| IBIS file stm32mp157xaa_lfbga448.ibs
[IBIS ver]   4.2
[File name]   stm32mp157xaa_lfbga448.ibs
[File Rev]   2.2
|   rev 2.0: better accuracy
[Date]   07-07-2026
[Source]   Data Created at STMicroelectronics
[Disclaimer]  This information is for modeling purpose only and is
   not guaranted.
   The information is subject to change without notice.
[Copyright]   Copyright 2026 STMicroelectronics Inc.
|   Component stm32mp157xaa_lfbga448
[Component] stm32mp157xaa_lfbga448
[Manufacturer] STMicroelectronics
[Package]
| variable   typ   min   max
R_pkg  6.18E-01  2.42E-01  9.67E-01
L_pkg  3.72E-09  1.45E-09  5.83E-09
C_pkg  1.34E-12  1.04E-12  5.48E-12
[Pin] signal_name model_name
A1 VSS GND
A10 PE3 io8_ft_hslv
A11 PA9 io8_ft_hslv
A12 PB3 io8_ft_hslv
A13 PB14 io8_ft_hslv
A14 VDD POWER
A15 DNU nc
A16 DNU nc
A17 DNU nc
A18 VDD1V2_Unused POWER
A19 VSS GND
A20 DDR_DQ20 PDDRIO_PAD
A21 DDR_DQ23 PDDRIO_PAD
A22 VSS GND
A2 PH5 io8_ft_i2c
A3 PH4 io8_ft_i2c
A4 PE13 io8_ft_hslv
A5 PK6 io8_ft_hslv
A6 PK4 io8_ft
A7 PJ13 io8_ft
A8 PD10 io8_ft_hslv
A9 PD5 io8_ft_hslv
AA1 PG13 io8_ft_hslv_et
AA10 PF7 io8_ft_hslv
AA11 PF6 io8_ft_hslv
AA12 BYPASS_REG1V8 nc
AA13 VSS_USBHS GND
AA14 USB_DM2 nc
AA15 USB_DP1 nc
AA16 VSS_USBHS GND
AA17 USB_RREF POWER
AA18 VSS GND
AA19 DDR_ATO nc
AA20 DDR_DQ29 PDDRIO_PAD
AA21 DDR_DQ28 PDDRIO_PAD
AA22 DDR_DQM3 PDDRIO_PAD
AA2 PG14 io8_ft_hslv_et
AA3 PA0 io8_ft_hslv
AA4 VSS GND
AA5 PB1 io8_ft_hslv
AA6 PC5 io8_ft_hslv
AA7 PB12 io8_ft_hslv_et
AA8 PB5 io8_ft_hslv_et
AA9 PG10 io8_ft_hslv
AB1 VSS GND
AB10 PF8 io8_ft_hslv
AB11 PF9 io8_ft_hslv
AB12 VDDA1V8_REG POWER
AB13 VDD3V3_USBHS POWER
AB14 USB_DP2 nc
AB15 USB_DM1 nc
AB16 VDD3V3_USBFS POWER
AB17 VDDA1V1_REG POWER
AB18 VSS GND
AB19 DDR_VREF POWER
AB20 DDR_DQ27 PDDRIO_PAD
AB21 DDR_DQ26 PDDRIO_PAD
AB22 VSS GND
AB2 PA2 io8_ft_hslv
AB3 PC1 io8_ft_hslv
AB4 PG4 io8_ft_hslv_et
AB5 PB0 io8_ft
AB6 PC4 io8_ft
AB7 PH2 io8_ft_hslv
AB8 PB8 io8_ft_et_i2c_hslv
AB9 PD11 io8_ft_hslv
B1 PH10 io8_ft
B10 PD1 io8_ft_i2c_hslv
B11 PD3 io8_ft_hslv
B12 PB15 io8_ft_hslv
B13 PA8 io8_ft_i2c_hslv
B14 VDDA1V8_Unused POWER
B15 DNU nc
B16 DNU nc
B17 DNU nc
B18 VDD1V2_Unused POWER
B19 VSS GND
B20 DDR_DQ19 PDDRIO_PAD
B21 DDR_DQ16 PDDRIO_PAD
B22 DDR_DQS2N PDIFF_PAD
B2 VSS GND
B3 PH11 io8_ft_i2c
B4 PE14 io8_ft_hslv
B5 PK7 io8_ft
B6 PK3 io8_ft
B7 PJ14 io8_ft
B8 PJ12 io8_ft
B9 PF1 io8_ft_i2c_hslv
C1 PH15 io8_ft
C10 PD0 io8_ft_i2c_hslv
C11 VSS GND
C12 PE5 io8_ft_hslv
C13 PB4 io8_ft_hslv
C14 VSS GND
C15 VSS GND
C16 VSS GND
C17 VSS GND
C18 VSS GND
C19 VSS GND
C20 VSS GND
C21 DDR_DQS2P PDIFF_PAD
C22 DDR_DQM2 PDDRIO_PAD
C2 PH14 io8_ft
C3 VSS GND
C4 PE15 io8_ft
C5 PE0 io8_ft_hslv
C6 PK5 io8_ft_hslv
C7 PJ15 io8_ft
C8 VSS GND
C9 PD4 io8_ft_hslv
D1 PI0 io8_ft
D10 PG15 io8_ft_i2c_hslv
D11 PG6 io8_ft_hslv
D12 PD2 io8_ft_hslv
D13 PC7 io8_ft_hslv
D14 PC9 io8_ft_i2c_hslv
D15 PC11 io8_ft_hslv
D16 JTDI io8_ft
D17 JTCK_SWCLK io8_ft
D18 VDD_PLL2 POWER
D19 VSS_PLL2 GND
D20 DDR_DQ22 PDDRIO_PAD
D21 DDR_DQ17 PDDRIO_PAD
D22 DDR_DQ18 PDDRIO_PAD
D2 PI14 io8_ft_hslv
D3 PH13 io8_ft
D4 VSS GND
D5 PE11 io8_ft
D6 PH8 io8_ft_i2c
D7 PE1 io8_ft
D8 PK0 io8_ft_hslv
D9 PF5 io8_ft_hslv
E1 PI2 io8_ft_hslv
E10 PF0 io8_ft_i2c_hslv
E11 PA15 io8_ft_hslv
E12 PC12 io8_ft_hslv
E13 PC6 io8_ft_hslv
E14 PC8 io8_ft_hslv
E15 NJTRST io8_ft_hslv
E16 JTDO_TRACESWO io8_ft_hslv
E17 JTMS_SWDIO io8_ft_hslv
E18 VDDQ_DDR POWER
E19 VSS GND
E20 DDR_DQ3 PDDRIO_PAD
E21 DDR_DQ0 PDDRIO_PAD
E22 DDR_DQ21 PDDRIO_PAD
E2 PI1 io8_ft_hslv
E3 PI3 io8_ft_hslv
E4 PE12 io8_ft_hslv
E5 VSS GND
E6 PH9 io8_ft
E7 PK1 io8_ft_hslv
E8 PK2 io8_ft_hslv
E9 PE6 io8_ft_hslv
F1 PI7 io8_ft
F10 PD7 io8_ft_i2c_hslv
F11 PB7 io8_ft_i2c_hslv
F12 PB9 io8_ft_i2c_hslv
F13 PF2 io8_ft_hslv
F14 PC10 io8_ft_hslv
F15 PE4 io8_ft_hslv
F16 VSS GND
F17 VDDQ_DDR POWER
F18 DDR_A7 PDDRIO_PAD
F19 DDR_RESETN PDDRIO_PAD
F20 VSS GND
F21 DDR_DQ1 PDDRIO_PAD
F2 PI5 io8_ft
F3 PI15 io8_ft
F4 PZ3 io8_ft_i2c
F5 PH12 io8_ft_i2c
F6 VSS GND
F7 VSS GND
F8 VSS GND
F9 PF4 io8_ft_hslv
G1 PZ4 io8_ft_i2c
G10 VSS GND
G12 VSS GND
G14 VSS GND
G16 VDDQ_DDR POWER
G17 VSS GND
G18 DDR_A13 PDDRIO_PAD
G19 DDR_DQ7 PDDRIO_PAD
G20 DDR_DQM0 PDDRIO_PAD
G21 DDR_DQS0N PDIFF_PAD
G22 DDR_DQS0P PDIFF_PAD
G2 PZ0 io8_ft_i2c_hslv
G3 PZ6 io8_ft_i2c
G4 VSS GND
G5 PI6 io8_ft
G6 VSS GND
G8 VSS GND
H1 PI13 io8_ft_hslv
H11 VDDCORE POWER
H13 VDDCORE POWER
H15 VDDCORE POWER
H17 VDDQ_DDR POWER
H18 DDR_A9 PDDRIO_PAD
H19 DDR_A5 PDDRIO_PAD
H20 DDR_DQ5 PDDRIO_PAD
H21 DDR_DQ2 PDDRIO_PAD
H22 DDR_DQ6 PDDRIO_PAD
H2 PI12 io8_ft_hslv
H3 PZ7 io8_ft_i2c
H4 PZ5 io8_ft_i2c
H5 PZ1 io8_ft_i2c_hslv
H6 PJ8 io8_ft_hslv
H7 VSS GND
H9 VDDCORE POWER
J1 PJ3 io8_ft_hslv
J10 VDDCORE POWER
J11 VSS GND
J12 VDDCORE POWER
J13 VSS GND
J14 VDDCORE POWER
J16 VDDQ_DDR POWER
J17 VSS GND
J18 DDR_A2 PDDRIO_PAD
J19 DDR_A3 PDDRIO_PAD
J20 VSS GND
J21 DDR_DQ4 PDDRIO_PAD
J2 PJ0 io8_ft_hslv
J3 PJ10 io8_ft_hslv
J4 PG12 io8_ft_hslv
J5 PI9 io8_ft
J6 PI4 io8_ft
J8 VDDCORE POWER
J9 VSS GND
K1 PJ5 io8_ft_hslv
K10 VSS GND
K11 VDDCORE POWER
K12 VSS GND
K13 VDDCORE POWER
K14 VSS GND
K15 VDDCORE POWER
K17 VDDQ_DDR POWER
K18 DDR_BA2 PDDRIO_PAD
K19 DDR_A0 PDDRIO_PAD
K20 DDR_BA0 PDDRIO_PAD
K21 DDR_DTO1 PDDRIO_PAD
K22 DDR_ZQ nc
K2 PJ4 io8_ft_hslv
K3 VSS GND
K4 PJ2 io8_ft_hslv
K5 PZ2 io8_ft_i2c_hslv
K6 PJ11 io8_ft_hslv
K7 VSS GND
K9 VDDCORE POWER
L1 PD15 io8_ft
L10 VDDCORE POWER
L11 VSS GND
L12 VDDCORE POWER
L13 VSS GND
L14 VDDCORE POWER
L16 VDDQ_DDR POWER
L17 VSS GND
L18 DDR_CSN PDDRIO_PAD
L19 VSS GND
L20 VSS GND
L21 DDR_ODT PDDRIO_PAD
L22 DDR_DTO0 PDDRIO_PAD
L2 PJ9 io8_ft_hslv
L3 PD6 io8_ft_hslv
L4 PJ7 io8_ft_hslv
L5 PJ6 io8_ft_hslv
L6 PJ1 io8_ft_hslv
L8 VDDCORE POWER
L9 VSS GND
M1 PD8 io8_ft
M10 VSS GND
M11 VDDCORE POWER
M12 VSS GND
M13 VDDCORE POWER
M14 VSS GND
M15 VDDCORE POWER
M17 VDDQ_DDR POWER
M18 DDR_A1 PDDRIO_PAD
M19 DDR_A15 PDDRIO_PAD
M20 DDR_RASN PDDRIO_PAD
M21 DDR_WEN PDDRIO_PAD
M22 DDR_CASN PDDRIO_PAD
M2 PD9 io8_ft
M3 PD14 io8_ft
M4 VBAT POWER
M5 VSS_PLL GND
M6 VDD_PLL POWER
M7 VSS GND
M9 VDD POWER
N1 PI8 io8_ft
N10 VDD POWER
N11 VSS GND
N12 VDDCORE POWER
N13 VSS GND
N14 VDDCORE POWER
N16 VDDQ_DDR POWER
N17 VSS GND
N18 DDR_A10 PDDRIO_PAD
N19 DDR_A12 PDDRIO_PAD
N20 DDR_CLKP PDDRIO_PAD
N21 DDR_CLKN PDDRIO_PAD
N22 DDR_DQ8 PDDRIO_PAD
N2 PC13 io8_ft
N3 BOOT0 io8_ft
N4 BOOT1 io8_ft
N5 VDD_ANA POWER
N6 VREFN GND
N8 VDD POWER
N9 VSS GND
P1 PC14_OSC32_IN io8_ft
P10 VSS GND
P11 VDD POWER
P12 VSS GND
P13 VDDCORE POWER
P14 VSS GND
P15 VDDCORE POWER
P17 VDDQ_DDR POWER
P18 DDR_A14 PDDRIO_PAD
P19 DDR_A11 PDDRIO_PAD
P20 VSS GND
P21 DDR_DQ10 PDDRIO_PAD
P2 PC15_OSC32_OUT io8_ft
P3 VSS GND
P4 BOOT2 io8_ft
P5 VSS_ANA GND
P6 VREF+ POWER
P7 VSS GND
P9 VDD POWER
R1 NRST_CORE isudqf
R10 VDD POWER
R12 VDD POWER
R14 VDDCORE POWER
R16 VDDQ_DDR POWER
R17 VSS GND
R18 DDR_BA1 PDDRIO_PAD
R19 DDR_CKE PDDRIO_PAD
R20 DDR_DQ13 PDDRIO_PAD
R21 DDR_DQ9 PDDRIO_PAD
R22 DDR_DQS1N PDIFF_PAD
|R2 NRST ioreset_ft_v33
R2 NRST nc
R3 PA14 io8_ft
R4 ANA0 nc
R5 VDDA POWER
R6 VSSA GND
R8 VSS GND
T1 PH0_OSC_IN io8_ft
T11 VSS GND
T13 VDD POWER
T15 VDDCORE POWER
T17 VDDQ_DDR POWER
T18 DDR_A4 PDDRIO_PAD
T19 VSS GND
T20 DDR_DQ11 PDDRIO_PAD
T21 DDR_DQM1 PDDRIO_PAD
T22 DDR_DQS1P PDIFF_PAD
T2 PH1_OSC_OUT io8_ft
T3 PI11 io8_ft
T4 PA3 io8_ft
T5 ANA1 nc
T6 VSSA GND
T7 VSS GND
T9 VSS GND
U1 PWR_LP io8_ft
U10 PC0 io8_ft_hslv
U11 PG11 io8_ft_hslv_et
U12 VDD POWER
U13 VSS GND
U14 VDD POWER
U15 VSS GND
U16 VDDQ_DDR POWER
U17 VSS GND
U18 DDR_A8 PDDRIO_PAD
U19 DDR_A6 PDDRIO_PAD
U20 VSS GND
U21 DDR_DQ14 PDDRIO_PAD
U2 PDR_ON_CORE isudqf
U3 PC3 io8_ft_hslv
U4 PG3 io8_ft_hslv_et
U5 PA5 io8_ft_hslv
U6 VSSA GND
U7 VSS GND
U8 PG5 io8_ft
U9 VDD_OTP POWER
V1 PWR_ON io8_ft
V10 PB13 io8_ft_hslv_et
V11 PH6 io8_ft_hslv
V12 PF10 io8_ft_hslv
V13 PB2 io8_ft_hslv
V14 PD13 io8_ft_i2c_hslv
V15 OTG_VBUS io8usb_vbus_otg20_ft
V16 VSS GND
V17 VDDQ_DDR POWER
V18 VSS GND
V19 VSS GND
V20 DDR_DQ12 PDDRIO_PAD
V21 DDR_DQ15 PDDRIO_PAD
V22 DDR_DQ24 PDDRIO_PAD
V2 PDR_ON isudqf
V3 PF3 io8_ft_hslv_et
V4 PA1 io8_ft_hslv
V5 VSS GND
V6 PA4 io8_ft
V7 PF14 io8_ft_i2c_hslv
V8 PF12 io8_ft_hslv
V9 PB10 io8_ft_hslv
W1 PI10 io8_ft
W10 PE7 io8_ft_hslv
W11 PE9 io8_ft_hslv
W12 PD12 io8_ft_i2c_hslv
W13 PB6 io8_ft_i2c_hslv
W14 PE10 io8_ft_hslv
W15 PG9 io8_ft_hslv
W16 PA12 io8_i2c_usb_lsfs_bcd_otg20_ft
W17 VSS GND
W18 VDDQ_DDR POWER
W19 VSS GND
W20 DDR_DQ25 PDDRIO_PAD
W21 DDR_DQ31 PDDRIO_PAD
W22 DDR_DQ30 PDDRIO_PAD
W2 PH7 io8_ft_i2c_hslv
W3 PA13 io8_ft
W4 PG2 io8_ft_hslv_et
W5 PG0 io8_ft_hslv_et
W6 PF15 io8_ft_i2c_hslv
W7 PF13 io8_ft_hslv
W8 PF11 io8_ft_hslv
W9 PA6 io8_ft_hslv
Y1 PC2 io8_ft_hslv_et
Y10 VSS GND
Y11 PG7 io8_ft_hslv
Y12 PE8 io8_ft_hslv
Y13 VSS_USBHS GND
Y14 VSS_USBHS GND
Y15 VSS_USBHS GND
Y16 PA11 io8_i2c_usb_lsfs_bcd_otg20_ft
Y17 PA10 io8usb_id_otg20_ft
Y18 VSS GND
Y19 VDDQ_DDR POWER
Y20 VSS GND
Y21 DDR_DQS3P PDIFF_PAD
Y22 DDR_DQS3N PDIFF_PAD
Y2 PE2 io8_ft_et_i2c_hslv
Y3 VSS GND
Y4 PG1 io8_ft_hslv_et
Y5 PB11 io8_ft_et_i2c_hslv
Y6 PH3 io8_ft_hslv
Y7 VSS GND
Y8 PG8 io8_ft_hslv_et
Y9 PA7 io8_ft_hslv
[Package Model]   500-lfbga-18x18-448-100mhz-181009
[Pin Mapping]   pulldown_ref   pullup_ref   | Comment
A1  VSS  nc
A2  VSS  VDD
A3  VSS  VDD
A4  VSS  VDD
A5  VSS  VDD
A6  VSS  VDD
A7  VSS  VDD
A8  VSS  VDD
A9  VSS  VDD
A10  VSS  VDD
A11  VSS  VDD
A12  VSS  VDD
A13  VSS  VDD
A14  nc  vdd
A15  nc  nc
A16  nc  nc
A17  nc  nc
A18  nc  vdd
A19  VSS  nc
A20  VSS  VDDQ_DDR
A21  VSS  VDDQ_DDR
A22  VSS  nc
AA1  VSS  VDD
AA2  VSS  VDD
AA3  VSS  VDD
AA4  VSS  nc
AA5  VSS  VDD
AA6  VSS  VDD
AA7  VSS  VDD
AA8  VSS  VDD
AA9  VSS  VDD
AA10  VSS  VDD
AA11  VSS  VDD
AA12  nc   nc
AA13  VSS_USBHS  nc
AA14  nc  nc
AA15  nc  nc
AA16  VSS_USBHS  nc
AA17  nc  VDD3V3_USBFS
AA18  VSS  nc
AA19  nc  nc
AA20  VSS  VDDQ_DDR
AA21  VSS  VDDQ_DDR
AA22  VSS  VDDQ_DDR
AB1  VSS  nc
AB2  VSS  VDD
AB3  VSS  VDD
AB4  VSS  VDD
AB5  VSS  VDD
AB6  VSS  VDD
AB7  VSS  VDD
AB8  VSS  VDD
AB9  VSS  VDD
AB10  VSS  VDD
AB11  VSS  VDD
AB12  nc  VDD3V3_USBFS
AB13  nc  vddusbhs
AB14  nc  nc
AB15  nc  nc
AB16  nc  VDD3V3_USBFS
AB17  nc  VDDA1V1_REG
AB18  VSS  nc
AB19  nc   VDDQ_DDR
AB20  VSS  VDDQ_DDR
AB21  VSS  VDDQ_DDR
AB22  VSS  nc
B1  VSS  VDD
B2  VSS  nc
B3  VSS  VDD
B4  VSS  VDD
B5  VSS  VDD
B6  VSS  VDD
B7  VSS  VDD
B8  VSS  VDD
B9  VSS  VDD
B10  VSS  VDD
B11  VSS  VDD
B12  VSS  VDD
B13  VSS  VDD
B14  nc  vdda
B15  nc  nc
B16  nc  nc
B17  nc  nc
B18  nc  VDD1V2_Unused
B19  VSS  nc
B20  VSS  VDDQ_DDR
B21  VSS  VDDQ_DDR
B22  VSS  VDDQ_DDR
C1  VSS  VDD
C2  VSS  VDD
C3  VSS  nc
C4  VSS  VDD
C5  VSS  VDD
C6  VSS  VDD
C7  VSS  VDD
C8  VSS  nc
C9  VSS  VDD
C10  VSS  VDD
C11  VSS  nc
C12  VSS  VDD
C13  VSS  VDD
C14  VSS  nc
C15  VSS  nc
C16  VSS  nc
C17  VSS  nc
C18  VSS  nc
C19  VSS  nc
C20  VSS  nc
C21  VSS  VDDQ_DDR
C22  VSS  VDDQ_DDR
D1  VSS  VDD
D2  VSS  VDD
D3  VSS  VDD
D4  VSS  nc
D5  VSS  VDD
D6  VSS  VDD
D7  VSS  VDD
D8  VSS  VDD
D9  VSS  VDD
D10  VSS  VDD
D11  VSS  VDD
D12  VSS  VDD
D13  VSS  VDD
D14  VSS  VDD
D15  VSS  VDD
D16  VSS  VDD
D17  VSS  VDD
D18  nc  VDD
D19  VSS  nc
D20  VSS  VDDQ_DDR
D21  VSS  VDDQ_DDR
D22  VSS  VDDQ_DDR
E1  VSS  VDD
E2  VSS  VDD
E3  VSS  VDD
E4  VSS  VDD
E5  VSS  nc
E6  VSS  VDD
E7  VSS  VDD
E8  VSS  VDD
E9  VSS  VDD
E10  VSS  VDD
E11  VSS  VDD
E12  VSS  VDD
E13  VSS  VDD
E14  VSS  VDD
E15  VSS  VDD
E16  VSS  VDD
E17  VSS  VDD
E18  nc  VDDQ_DDR
E19  VSS  nc
E20  VSS  VDDQ_DDR
E21  VSS  VDDQ_DDR
E22  VSS  VDDQ_DDR
F1  VSS  VDD
F2  VSS  VDD
F3  VSS  VDD
F4  VSS  VDD
F5  VSS  VDD
F6  VSS  nc
F7  VSS  nc
F8  VSS  nc
F9  VSS  VDD
F10  VSS  VDD
F11  VSS  VDD
F12  VSS  VDD
F13  VSS  VDD
F14  VSS  VDD
F15  VSS  VDD
F16  VSS  nc
F17  nc  VDDQ_DDR
F18  VSS  VDDQ_DDR
F19  VSS  VDDQ_DDR
F20  VSS  nc
F21  VSS  VDDQ_DDR
G1  VSS  VDD
G2  VSS  VDD
G3  VSS  VDD
G4  VSS  nc
G5  VSS  VDD
G6  VSS  nc
G8  VSS  nc
G10  VSS  nc
G12  VSS  nc
G14  VSS  nc
G16  nc  VDDQ_DDR
G17  VSS  nc
G18  VSS  VDDQ_DDR
G19  VSS  VDDQ_DDR
G20  VSS  VDDQ_DDR
G21  VSS  VDDQ_DDR
G22  VSS  VDDQ_DDR
H1  VSS  VDD
H2  VSS  VDD
H3  VSS  VDD
H4  VSS  VDD
H5  VSS  VDD
H6  VSS  VDD
H7  VSS  nc
H9  nc  VDDCORE
H11  nc  VDDCORE
H13  nc  VDDCORE
H15  nc  VDDCORE
H17  nc  VDDQ_DDR
H18  VSS  VDDQ_DDR
H19  VSS  VDDQ_DDR
H20  VSS  VDDQ_DDR
H21  VSS  VDDQ_DDR
H22  VSS  VDDQ_DDR
J1  VSS  VDD
J2  VSS  VDD
J3  VSS  VDD
J4  VSS  VDD
J5  VSS  VDD
J6  VSS  VDD
J8  nc  VDDCORE
J9  VSS  nc
J10  nc  VDDCORE
J11  VSS  nc
J12  nc  VDDCORE
J13  VSS  nc
J14  nc  VDDCORE
J16  nc  VDDQ_DDR
J17  VSS  nc
J18  VSS  VDDQ_DDR
J19  VSS  VDDQ_DDR
J20  VSS  nc
J21  VSS  VDDQ_DDR
K1  VSS  VDD
K2  VSS  VDD
K3  VSS  nc
K4  VSS  VDD
K5  VSS  VDD
K6  VSS  VDD
K7  VSS  nc
K9  nc  VDDCORE
K10  VSS  nc
K11  nc  VDDCORE
K12  VSS  nc
K13  nc  VDDCORE
K14  VSS  nc
K15  nc  VDDCORE
K17  nc  VDDQ_DDR
K18  VSS  VDDQ_DDR
K19  VSS  VDDQ_DDR
K20  VSS  VDDQ_DDR
K21  VSS  VDDQ_DDR
K22  nc  nc
L1  VSS  VDD
L2  VSS  VDD
L3  VSS  VDD
L4  VSS  VDD
L5  VSS  VDD
L6  VSS  VDD
L8  nc  VDDCORE
L9  VSS  nc
L10  nc  VDDCORE
L11  VSS  nc
L12  nc  VDDCORE
L13  VSS  nc
L14  nc  VDDCORE
L16  nc  VDDQ_DDR
L17  VSS  nc
L18  VSS  VDDQ_DDR
L19  VSS  nc
L20  VSS  nc
L21  VSS  VDDQ_DDR
L22  VSS  VDDQ_DDR
M1  VSS  VDD
M2  VSS  VDD
M3  VSS  VDD
M4  nc  VDD_sw
M5  VSS  nc
M6  nc  VDD
M7  VSS  nc
M9  nc  VDD
M10  VSS  nc
M11  nc  VDDCORE
M12  VSS  nc
M13  nc  VDDCORE
M14  VSS  nc
M15  nc  VDDCORE
M17  nc  VDDQ_DDR
M18  VSS  VDDQ_DDR
M19  VSS  VDDQ_DDR
M20  VSS  VDDQ_DDR
M21  VSS  VDDQ_DDR
M22  VSS  VDDQ_DDR
N1  nc  nc
N2  nc  nc
N3  VSS  VDD
N4  VSS  VDD
N5  nc  VDD
N6  VSS  nc
N8  nc  VDD
N9  VSS  nc
N10  nc  VDD
N11  VSS  nc
N12  nc  VDDCORE
N13  VSS  nc
N14  nc  VDDCORE
N16  nc  VDDQ_DDR
N17  VSS  nc
N18  VSS  VDDQ_DDR
N19  VSS  VDDQ_DDR
N20  VSS  VDDQ_DDR
N21  VSS  VDDQ_DDR
N22  VSS  VDDQ_DDR
P1  nc  nc
P2  nc  nc
P3  VSS  nc
P4  VSS  VDD
P5  VSS  nc
P6  nc  VDD
P7  VSS  nc
P9  nc  VDD
P10  VSS  nc
P11  nc  VDD
P12  VSS  nc
P13  nc  VDDCORE
P14  VSS  nc
P15  nc  VDDCORE
P17  nc  VDDQ_DDR
P18  VSS  VDDQ_DDR
P19  VSS  VDDQ_DDR
P20  VSS  nc
P21  VSS  VDDQ_DDR
R1  nc  nc
R2  nc  nc
R3  VSS  VDD
R4  nc  nc
R5  nc  VDD
R6  VSS  nc
R8  VSS  nc
R10  nc  VDD
R12  nc  VDD
R14  nc  VDDCORE
R16  nc  VDDQ_DDR
R17  VSS  nc
R18  VSS  VDDQ_DDR
R19  VSS  VDDQ_DDR
R20  VSS  VDDQ_DDR
R21  VSS  VDDQ_DDR
R22  VSS  VDDQ_DDR
T1  VSS  VDD
T2  VSS  VDD
T3  VSS  VDD
T4  VSS  VDD
T5  nc  nc
T6  VSS  nc
T7  VSS  nc
T9  VSS  nc
T11  VSS  nc
T13  nc  VDD
T15  nc  VDDCORE
T17  nc  VDDQ_DDR
T18  VSS  VDDQ_DDR
T19  VSS  nc
T20  VSS  VDDQ_DDR
T21  VSS  VDDQ_DDR
T22  VSS  VDDQ_DDR
U1  VSS  VDD
U2  nc  nc
U3  VSS  VDD
U4  VSS  VDD
U5  VSS  VDD
U6  VSS  nc
U7  VSS  nc
U8  VSS  VDD
U9  nc  VDD
U10  VSS  VDD
U11  VSS  VDD
U12  nc  VDD
U13  VSS  nc
U14  nc  VDD
U15  VSS  nc
U16  nc  VDDQ_DDR
U17  VSS  nc
U18  VSS  VDDQ_DDR
U19  VSS  VDDQ_DDR
U20  VSS  nc
U21  VSS  VDDQ_DDR
V1  VSS  VDD
V2  nc  nc
V3  VSS  VDD
V4  VSS  VDD
V5  VSS  nc
V6  VSS  VDD
V7  VSS  VDD
V8  VSS  VDD
V9  VSS  VDD
V10  VSS  VDD
V11  VSS  VDD
V12  VSS  VDD
V13  VSS  VDD
V14  VSS  VDD
V15  VSS  VDD3V3_USBFS  | Depending on IO usage
| V15  VSS  VDD  | Depending on IO usage
V16  VSS  nc
V17  nc  VDDQ_DDR
V18  VSS  nc
V19  VSS  nc
V20  VSS  VDDQ_DDR
V21  VSS  VDDQ_DDR
V22  VSS  VDDQ_DDR
W1  VSS  VDD
W2  VSS  VDD
W3  VSS  VDD
W4  VSS  VDD
W5  VSS  VDD
W6  VSS  VDD
W7  VSS  VDD
W8  VSS  VDD
W9  VSS  VDD
W10  VSS  VDD
W11  VSS  VDD
W12  VSS  VDD
W13  VSS  VDD
W14  VSS  VDD
W15  VSS  VDD
W16  VSS  VDD3V3_USBFS  | Depending on IO usage
| W16  VSS  VDD  | Depending on IO usage
W17  VSS  nc
W18  nc  VDDQ_DDR
W19  VSS  nc
W20  VSS  VDDQ_DDR
W21  VSS  VDDQ_DDR
W22  VSS  VDDQ_DDR
Y1  VSS  VDD
Y2  VSS  VDD
Y3  VSS  nc
Y4  VSS  VDD
Y5  VSS  VDD
Y6  VSS  VDD
Y7  VSS  nc
Y8  VSS  VDD
Y9  VSS  VDD
Y10  VSS  nc
Y11  VSS  VDD
Y12  VSS  VDD
Y13  VSS_USBHS  nc
Y14  VSS_USBHS  nc
Y15  VSS_USBHS  nc
Y16  VSS  VDD3V3_USBFS  | Depending on IO usage
| Y16  VSS  VDD  | Depending on IO usage
Y17  VSS  VDD3V3_USBFS  | Depending on IO usage
| Y17  VSS  VDD  | Depending on IO usage
Y18  VSS  nc
Y19  nc  VDDQ_DDR
Y20  VSS  nc
Y21  VSS  VDDQ_DDR
Y22  VSS  VDDQ_DDR
|**********************DIFF PIN*********************************************
[Diff_pin]   inv_pin   vdiff   tdelay_typ   tdelay_min   tdelay_max
   N20   N21   0.320V   0ns   NA   NA   |CK
   G22   G21   0.320V   0ns   NA   NA   |DQS0
   T22   R22   0.320V   0ns   NA   NA   |DQS1
   C21   B22   0.320V   0ns   NA   NA   |DQS2
   Y21   Y22   0.320V   0ns   NA   NA   |DQS3
[Model Selector] io8usb_id_otg20_ft
io8_ft_ls_1v2   "GPIO - 5V tolerant - 1.2V range - Low speed"
io8_ft_ms_1v2   "GPIO - 5V tolerant - 1.2V range - Med speed"
io8_ft_hs_1v2   "GPIO - 5V tolerant - 1.2V range - High speed"
io8_ft_fs_1v2   "GPIO - 5V tolerant - 1.2V range - Fast speed"
io8_ft_hs_1v8   "GPIO - 5V tolerant - 1.8V range - High speed"
io8_ft_fs_1v8   "GPIO - 5V tolerant - 1.8V range - Fast speed"
io8_ft_ms_1v8   "GPIO - 5V tolerant - 1.8V range - Med speed"
io8_ft_ls_1v8   "GPIO - 5V tolerant - 1.8V range - Low speed"
io8_ft_hs_3v3   "GPIO - 5V tolerant - 3.3V range - High speed"
io8_ft_fs_3v3   "GPIO - 5V tolerant - 3.3V range - Fast speed"
io8_ft_ms_3v3   "GPIO - 5V tolerant - 3.3V range - Med speed"
io8_ft_ls_3v3   "GPIO - 5V tolerant - 3.3V range - Low speed"
[Model Selector] io8usb_vbus_otg20_ft
io8_ft_ls_1v2   "GPIO - 5V tolerant - 1.2V range - Low speed"
io8_ft_ms_1v2   "GPIO - 5V tolerant - 1.2V range - Med speed"
io8_ft_hs_1v2   "GPIO - 5V tolerant - 1.2V range - High speed"
io8_ft_fs_1v2   "GPIO - 5V tolerant - 1.2V range - Fast speed"
io8_ft_hs_1v8   "GPIO - 5V tolerant - 1.8V range - High speed"
io8_ft_fs_1v8   "GPIO - 5V tolerant - 1.8V range - Fast speed"
io8_ft_ms_1v8   "GPIO - 5V tolerant - 1.8V range - Med speed"
io8_ft_ls_1v8   "GPIO - 5V tolerant - 1.8V range - Low speed"
io8_ft_hs_3v3   "GPIO - 5V tolerant - 3.3V range - High speed"
io8_ft_fs_3v3   "GPIO - 5V tolerant - 3.3V range - Fast speed"
io8_ft_ms_3v3   "GPIO - 5V tolerant - 3.3V range - Med speed"
io8_ft_ls_3v3   "GPIO - 5V tolerant - 3.3V range - Low speed"
[Model Selector] io8_ft
io8_ft_ls_1v2   "GPIO - 5V tolerant - 1.2V range - Low speed"
io8_ft_ms_1v2   "GPIO - 5V tolerant - 1.2V range - Med speed"
io8_ft_hs_1v2   "GPIO - 5V tolerant - 1.2V range - High speed"
io8_ft_fs_1v2   "GPIO - 5V tolerant - 1.2V range - Fast speed"
io8_ft_hs_1v8   "GPIO - 5V tolerant - 1.8V range - High speed"
io8_ft_fs_1v8   "GPIO - 5V tolerant - 1.8V range - Fast speed"
io8_ft_ms_1v8   "GPIO - 5V tolerant - 1.8V range - Med speed"
io8_ft_ls_1v8   "GPIO - 5V tolerant - 1.8V range - Low speed"
io8_ft_hs_3v3   "GPIO - 5V tolerant - 3.3V range - High speed"
io8_ft_fs_3v3   "GPIO - 5V tolerant - 3.3V range - Fast speed"
io8_ft_ms_3v3   "GPIO - 5V tolerant - 3.3V range - Med speed"
io8_ft_ls_3v3   "GPIO - 5V tolerant - 3.3V range - Low speed"
[Model Selector] io8_ft_hslv
io8_ft_ls_1v2   "GPIO - 5V tolerant - 1.2V range - Low speed"
io8_ft_ms_1v2   "GPIO - 5V tolerant - 1.2V range - Med speed"
io8_ft_hs_1v2   "GPIO - 5V tolerant - 1.2V range - High speed"
io8_ft_fs_1v2   "GPIO - 5V tolerant - 1.2V range - Fast speed"
io8_ft_hs_1v8   "GPIO - 5V tolerant - 1.8V range - High speed"
io8_ft_fs_1v8   "GPIO - 5V tolerant - 1.8V range - Fast speed"
io8_ft_ms_1v8   "GPIO - 5V tolerant - 1.8V range - Med speed"
io8_ft_ls_1v8   "GPIO - 5V tolerant - 1.8V range - Low speed"
io8_ft_hs_3v3   "GPIO - 5V tolerant - 3.3V range - High speed"
io8_ft_fs_3v3   "GPIO - 5V tolerant - 3.3V range - Fast speed"
io8_ft_ms_3v3   "GPIO - 5V tolerant - 3.3V range - Med speed"
io8_ft_ls_3v3   "GPIO - 5V tolerant - 3.3V range - Low speed"
io8_ft_hslv_hs_1v2   "GPIO - hslv opt - 5V tolerant - 1.2V range - High speed"
io8_ft_hslv_fs_1v2   "GPIO - hslv opt - 5V tolerant - 1.2V range - Fast speed"
io8_ft_hslv_ms_1v2   "GPIO - hslv opt - 5V tolerant - 1.2V range - Med speed"
io8_ft_hslv_ls_1v2   "GPIO - hslv opt - 5V tolerant - 1.2V range - Low speed"
io8_ft_hslv_hs_1v8   "GPIO - hslv opt - 5V tolerant - 1.8V range - High speed"
io8_ft_hslv_fs_1v8   "GPIO - hslv opt - 5V tolerant - 1.8V range - Fast speed"
io8_ft_hslv_ms_1v8   "GPIO - hslv opt - 5V tolerant - 1.8V range - Med speed"
io8_ft_hslv_ls_1v8   "GPIO - hslv opt - 5V tolerant - 1.8V range - Low speed"
io8_ft_hslv_hs_2v5   "GPIO - hslv opt - 5V tolerant - 2.5V range - High speed"
io8_ft_hslv_fs_2v5   "GPIO - hslv opt - 5V tolerant - 2.5V range - Fast speed"
io8_ft_hslv_ms_2v5   "GPIO - hslv opt - 5V tolerant - 2.5V range - Med speed"
io8_ft_hslv_ls_2v5   "GPIO - hslv opt - 5V tolerant - 2.5V range - Low speed"
[Model Selector] io8_ft_hslv_et
io8_ft_et_ls_1v2   "GPIO - Ethernet - 5V tol - 1.2V range - Low speed"
io8_ft_et_ms_1v2   "GPIO - Ethernet - 5V tol - 1.2V range - Med speed"
io8_ft_et_hs_1v2   "GPIO - Ethernet - 5V tol - 1.2V range - High speed"
io8_ft_et_fs_1v2   "GPIO - Ethernet - 5V tol - 1.2V range - Fast speed"
io8_ft_et_hs_1v8   "GPIO - Ethernet - 5V tol - 1.8V range - High speed"
io8_ft_et_fs_1v8   "GPIO - Ethernet - 5V tol - 1.8V range - Fast speed"
io8_ft_et_ms_1v8   "GPIO - Ethernet - 5V tol - 1.8V range - Med speed"
io8_ft_et_ls_1v8   "GPIO - Ethernet - 5V tol - 1.8V range - Low speed"
io8_ft_et_hs_3v3   "GPIO - Ethernet - 5V tol - 3.3V range - High speed"
io8_ft_et_fs_3v3   "GPIO - Ethernet - 5V tol - 3.3V range - Fast speed"
io8_ft_et_ms_3v3   "GPIO - Ethernet - 5V tol - 3.3V range - Med speed"
io8_ft_et_ls_3v3   "GPIO - Ethernet - 5V tol - 3.3V range - Low speed"
io8_ft_et_hslv_ls_1v2   "GPIO - hslv opt - Ethernet - 5V tol - 1.2V range - Low speed"
io8_ft_et_hslv_hs_1v2   "GPIO - hslv opt - Ethernet - 5V tol - 1.2V range - High speed"
io8_ft_et_hslv_fs_1v2   "GPIO - hslv opt - Ethernet - 5V tol - 1.2V range - Fast speed"
io8_ft_et_hslv_ms_1v2   "GPIO - hslv opt - Ethernet - 5V tol - 1.2V range - Med speed"
io8_ft_et_hslv_ls_1v8   "GPIO - hslv opt - Ethernet - 5V tol - 1.8V range - Low speed"
io8_ft_et_hslv_hs_1v8   "GPIO - hslv opt - Ethernet - 5V tol - 1.8V range - High speed"
io8_ft_et_hslv_fs_1v8   "GPIO - hslv opt - Ethernet - 5V tol - 1.2V range - Fast speed"
io8_ft_et_hslv_ms_1v8   "GPIO - hslv opt - Ethernet - 5V tol - 1.8V range - Med speed"
io8_ft_et_hslv_hs_2v5   "GPIO - hslv opt - Ethernet - 5V tol - 2.5V range - High speed"
io8_ft_et_hslv_fs_2v5   "GPIO - hslv opt - Ethernet - 5V tol - 2.5V range - Fast speed"
io8_ft_et_hslv_ms_2v5   "GPIO - hslv opt - Ethernet - 5V tol - 2.5V range - Med speed"
io8_ft_et_hslv_ls_2v5   "GPIO - hslv opt - Ethernet - 5V tol - 2.5V range - Low speed"
[Model Selector] io8_ft_et_i2c_hslv
io8_ft_et_ls_1v2   "GPIO - 5V tol - 1.2V range - Low speed"
io8_ft_et_ms_1v2   "GPIO - 5V tol - 1.2V range - Med speed"
io8_ft_et_hs_1v2   "GPIO - 5V tol - 1.2V range - High speed"
io8_ft_et_fs_1v2   "GPIO - 5V tol - 1.2V range - Fast speed"
io8_ft_et_hs_1v8   "GPIO - 5V tol - 1.8V range - High speed"
io8_ft_et_fs_1v8   "GPIO - 5V tol - 1.8V range - Fast speed"
io8_ft_et_ms_1v8   "GPIO - 5V tol - 1.8V range - Med speed"
io8_ft_et_ls_1v8   "GPIO - 5V tol - 1.8V range - Low speed"
io8_ft_et_hs_3v3   "GPIO - 5V tol - 3.3V range - High speed"
io8_ft_et_fs_3v3   "GPIO - 5V tol - 3.3V range - Fast speed"
io8_ft_et_ms_3v3   "GPIO - 5V tol - 3.3V range - Med speed"
io8_ft_et_ls_3v3   "GPIO - 5V tol - 3.3V range - Low speed"
io8_ft_et_hslv_ls_1v2   "GPIO - hslv opt -Ethernet - 5V tol - 1.2V range - Low speed"
io8_ft_et_hslv_hs_1v2   "GPIO - hslv opt -Ethernet - 5V tol - 1.2V range - High speed"
io8_ft_et_hslv_fs_1v2   "GPIO - hslv opt -Ethernet - 5V tol - 1.2V range - Fast speed"
io8_ft_et_hslv_ms_1v2   "GPIO - hslv opt -Ethernet - 5V tol - 1.2V range - Med speed"
io8_ft_et_hslv_ls_1v8   "GPIO - hslv opt -Ethernet - 5V tol - 1.8V range - Low speed"
io8_ft_et_hslv_hs_1v8   "GPIO - hslv opt -Ethernet - 5V tol - 1.8V range - High speed"
io8_ft_et_hslv_fs_1v8   "GPIO - hslv opt -Ethernet - 5V tol - 1.2V range - Fast speed"
io8_ft_et_hslv_ms_1v8   "GPIO - hslv opt -Ethernet - 5V tol - 1.8V range - Med speed"
io8_ft_et_hslv_hs_2v5   "GPIO - hslv opt -Ethernet - 5V tol - 2.5V range - High speed"
io8_ft_et_hslv_fs_2v5   "GPIO - hslv opt  -Ethernet- 5V tol - 2.5V range - Fast speed"
io8_ft_et_hslv_ms_2v5   "GPIO - hslv opt -Ethernet - 5V tol - 2.5V range - Med speed"
io8_ft_et_hslv_ls_2v5   "GPIO - hslv opt -Ethernet - 5V tol - 2.5V range - Low speed"
io8_ft_i2c_1v2   "GPIO - 5V tolerant - 1.2V range - Open drain"
io8_ft_i2c_1v8   "GPIO - 5V tolerant - 1.8V range - Open drain"
io8_ft_i2c_3v3   "GPIO - 5V tolerant - 3.3V range - Open drain"
io8_ft_i2c_hslv_1v2   "GPIO - hslv opt - 5V tolerant - 1.2V range - Open drain"
io8_ft_i2c_hslv_1v8   "GPIO - hslv opt - 5V tolerant - 1.8V range - Open drain"
io8_ft_i2c_hslv_2v5   "GPIO - hslv opt - 5V tolerant - 2.5V range - Open drain"
io8_ft_hslv_hs_1v2   "GPIO - hslv opt - 5V tolerant - 1.2V range - High speed"
io8_ft_hslv_fs_1v2   "GPIO - hslv opt - 5V tolerant - 1.2V range - Fast speed"
io8_ft_hslv_ms_1v2   "GPIO - hslv opt - 5V tolerant - 1.2V range - Med speed"
io8_ft_hslv_ls_1v2   "GPIO - hslv opt - 5V tolerant - 1.2V range - Low speed"
io8_ft_hslv_hs_1v8   "GPIO - hslv opt - 5V tolerant - 1.8V range - High speed"
io8_ft_hslv_fs_1v8   "GPIO - hslv opt - 5V tolerant - 1.8V range - Fast speed"
io8_ft_hslv_ms_1v8   "GPIO - hslv opt - 5V tolerant - 1.8V range - Med speed"
io8_ft_hslv_ls_1v8   "GPIO - hslv opt - 5V tolerant - 1.8V range - Low speed"
io8_ft_hslv_hs_2v5   "GPIO - hslv opt - 5V tolerant - 2.5V range - High speed"
io8_ft_hslv_fs_2v5   "GPIO - hslv opt - 5V tolerant - 2.5V range - Fast speed"
io8_ft_hslv_ms_2v5   "GPIO - hslv opt - 5V tolerant - 2.5V range - Med speed"
io8_ft_hslv_ls_2v5   "GPIO - hslv opt - 5V tolerant - 2.5V range - Low speed"
[Model Selector] io8_ft_i2c
io8_ft_ls_1v2   "GPIO - 5V tolerant - 1.2V range - Low speed"
io8_ft_ms_1v2   "GPIO - 5V tolerant - 1.2V range - Med speed"
io8_ft_hs_1v2   "GPIO - 5V tolerant - 1.2V range - High speed"
io8_ft_fs_1v2   "GPIO - 5V tolerant - 1.2V range - Fast speed"
io8_ft_hs_1v8   "GPIO - 5V tolerant - 1.8V range - High speed"
io8_ft_fs_1v8   "GPIO - 5V tolerant - 1.8V range - Fast speed"
io8_ft_ms_1v8   "GPIO - 5V tolerant - 1.8V range - Med speed"
io8_ft_ls_1v8   "GPIO - 5V tolerant - 1.8V range - Low speed"
io8_ft_hs_3v3   "GPIO - 5V tolerant - 3.3V range - High speed"
io8_ft_fs_3v3   "GPIO - 5V tolerant - 3.3V range - Fast speed"
io8_ft_ms_3v3   "GPIO - 5V tolerant - 3.3V range - Med speed"
io8_ft_ls_3v3   "GPIO - 5V tolerant - 3.3V range - Low speed"
io8_ft_i2c_1v2   "GPIO - 5V tolerant - 1.2V range - Open drain"
io8_ft_i2c_1v8   "GPIO - 5V tolerant - 1.8V range - Open drain"
io8_ft_i2c_3v3   "GPIO - 5V tolerant - 3.3V range - Open drain"
[Model Selector] io8_ft_i2c_hslv
io8_ft_ls_1v2   "GPIO - 5V tolerant - 1.2V range - Low speed"
io8_ft_ms_1v2   "GPIO - 5V tolerant - 1.2V range - Med speed"
io8_ft_hs_1v2   "GPIO - 5V tolerant - 1.2V range - High speed"
io8_ft_fs_1v2   "GPIO - 5V tolerant - 1.2V range - Fast speed"
io8_ft_hs_1v8   "GPIO - 5V tolerant - 1.8V range - High speed"
io8_ft_fs_1v8   "GPIO - 5V tolerant - 1.8V range - Fast speed"
io8_ft_ms_1v8   "GPIO - 5V tolerant - 1.8V range - Med speed"
io8_ft_ls_1v8   "GPIO - 5V tolerant - 1.8V range - Low speed"
io8_ft_hs_3v3   "GPIO - 5V tolerant - 3.3V range - High speed"
io8_ft_fs_3v3   "GPIO - 5V tolerant - 3.3V range - Fast speed"
io8_ft_ms_3v3   "GPIO - 5V tolerant - 3.3V range - Med speed"
io8_ft_ls_3v3   "GPIO - 5V tolerant - 3.3V range - Low speed"
io8_ft_hslv_hs_1v2   "GPIO - hslv opt - 5V tolerant - 1.2V range - High speed"
io8_ft_hslv_fs_1v2   "GPIO - hslv opt - 5V tolerant - 1.2V range - Fast speed"
io8_ft_hslv_ms_1v2   "GPIO - hslv opt - 5V tolerant - 1.2V range - Med speed"
io8_ft_hslv_ls_1v2   "GPIO - hslv opt - 5V tolerant - 1.2V range - Low speed"
io8_ft_hslv_hs_1v8   "GPIO - hslv opt - 5V tolerant - 1.8V range - High speed"
io8_ft_hslv_fs_1v8   "GPIO - hslv opt - 5V tolerant - 1.8V range - Fast speed"
io8_ft_hslv_ms_1v8   "GPIO - hslv opt - 5V tolerant - 1.8V range - Med speed"
io8_ft_hslv_ls_1v8   "GPIO - hslv opt - 5V tolerant - 1.8V range - Low speed"
io8_ft_hslv_hs_2v5   "GPIO - hslv opt - 5V tolerant - 2.5V range - High speed"
io8_ft_hslv_fs_2v5   "GPIO - hslv opt - 5V tolerant - 2.5V range - Fast speed"
io8_ft_hslv_ms_2v5   "GPIO - hslv opt - 5V tolerant - 2.5V range - Med speed"
io8_ft_hslv_ls_2v5   "GPIO - hslv opt - 5V tolerant - 2.5V range - Low speed"
io8_ft_i2c_1v2   "GPIO - 5V tolerant - 1.2V range - Open drain"
io8_ft_i2c_1v8   "GPIO - 5V tolerant - 1.8V range - Open drain"
io8_ft_i2c_3v3   "GPIO - 5V tolerant - 3.3V range - Open drain"
io8_ft_i2c_hslv_1v2   "GPIO - hslv opt - 5V tolerant - 1.2V range - Open drain"
io8_ft_i2c_hslv_1v8   "GPIO - hslv opt - 5V tolerant - 1.8V range - Open drain"
io8_ft_i2c_hslv_2v5   "GPIO - hslv opt - 5V tolerant - 2.5V range - Open drain"
[Model Selector] io8_i2c_usb_lsfs_bcd_otg20_ft
io8_ft_ls_1v2   "GPIO - 5V tolerant - 1.2V range - Low speed"
io8_ft_ms_1v2   "GPIO - 5V tolerant - 1.2V range - Med speed"
io8_ft_hs_1v2   "GPIO - 5V tolerant - 1.2V range - High speed"
io8_ft_fs_1v2   "GPIO - 5V tolerant - 1.2V range - Fast speed"
io8_ft_hs_1v8   "GPIO - 5V tolerant - 1.8V range - High speed"
io8_ft_fs_1v8   "GPIO - 5V tolerant - 1.8V range - Fast speed"
io8_ft_ms_1v8   "GPIO - 5V tolerant - 1.8V range - Med speed"
io8_ft_ls_1v8   "GPIO - 5V tolerant - 1.8V range - Low speed"
io8_ft_hs_3v3   "GPIO - 5V tolerant - 3.3V range - High speed"
io8_ft_fs_3v3   "GPIO - 5V tolerant - 3.3V range - Fast speed"
io8_ft_ms_3v3   "GPIO - 5V tolerant - 3.3V range - Med speed"
io8_ft_ls_3v3   "GPIO - 5V tolerant - 3.3V range - Low speed"
io8_ft_i2c_1v2   "GPIO - 5V tolerant - 1.2V range - Open drain"
io8_ft_i2c_1v8   "GPIO - 5V tolerant - 1.8V range - Open drain"
io8_ft_i2c_3v3   "GPIO - 5V tolerant - 3.3V range - Open drain"
io8usb_ft_hs_3v3   "USB full speed"
io8usb_ft_ls_3v3   "USB low speed"
[Model Selector] isudqf
isudqf_1v2   "Input Buffer - 5V tolerant - 1.2V range"
isudqf_1v8   "Input Buffer - 5V tolerant - 1.8V range"
isudqf_3v3   "Input Buffer - 5V tolerant - 3.3V range"
[Model Selector] PDIFF_PAD
MSD_D3RF2_18   DDR2 MSD_D3R_PDIFF Z0=18-Ohm
MSD_D3RF2_40   DDR2 MSD_D3R_PDIFF Z0=40-Ohm
MSD_D3RF2_48   DDR2 MSD_D3R_PDIFF Z0=48-Ohm
MSD_D3RF2_ODT150   DDR2 MSD_D3R_PDIFF cell 150-Ohm ODT Receiver
MSD_D3RF2_ODT50   DDR2 MSD_D3R_PDIFF cell 50-Ohm ODT Receiver
MSD_D3RF2_ODT75   DDR2 MSD_D3R_PDIFF cell 75-Ohm ODT Receiver
MSD_D3RF2_ODTOFF   DDR2 MSD_D3R_PDIFF cell ODT off Receiver
MSD_D3RF3_34   DDR3 MSD_D3R_PDIFF cell  Z0=34-Ohm
MSD_D3RF3_40   DDR3 MSD_D3R_PDIFF cell  Z0=40-Ohm
MSD_D3RF3_48   DDR3 MSD_D3R_PDIFF cell  Z0=48-Ohm
MSD_D3RF3L_34   DDR3L MSD_D3R_PDIFF cell  Z0=34-Ohm
MSD_D3RF3L_40   DDR3L MSD_D3R_PDIFF cell  Z0=40-Ohm
MSD_D3RF3L_48   DDR3L MSD_D3R_PDIFF cell  Z0=48-Ohm
MSD_D3RF3L_ODT120   DDR3L MSD_D3R_PDIFF cell 120-Ohm ODT Receiver
MSD_D3RF3L_ODT40   DDR3L MSD_D3R_PDIFF cell 40-Ohm ODT Receiver
MSD_D3RF3L_ODT60   DDR3L MSD_D3R_PDIFF cell 60-Ohm ODT Receiver
MSD_D3RF3L_ODTOFF   DDR3L MSD_D3R_PDIFF cell ODT off Receiver
MSD_D3RF3_ODT120   DDR3 MSD_D3R_PDIFF cell 120-Ohm ODT Receiver
MSD_D3RF3_ODT40   DDR3 MSD_D3R_PDIFF cell 40-Ohm ODT Receiver
MSD_D3RF3_ODT60   DDR3 MSD_D3R_PDIFF cell 60-Ohm ODT Receiver
MSD_D3RF3_ODTOFF   DDR3 MSD_D3R_PDIFF cell ODT off Receiver
MSD_D3RFL2_34   LPDDR2 MSD_D3R_PDIFF cell  Z0=34-Ohm
MSD_D3RFL2_40   LPDDR2 MSD_D3R_PDIFF cell  Z0=40-Ohm
MSD_D3RFL2_48   LPDDR2 MSD_D3R_PDIFF cell  Z0=48-Ohm
MSD_D3RFL2_60   LPDDR2 MSD_D3R_PDIFF cell  Z0=60-Ohm
MSD_D3RFL2_80   LPDDR2 MSD_D3R_PDIFF cell  Z0=80-Ohm
MSD_D3RFL2_ODTOFF   LPDDR2 MSD_D3R_PDIFF cell ODT off Receiver
MSD_D3RFL_48   LPDDR MSD_D3R_PDIFF cell  Z0=48-Ohm
MSD_D3RFL_ODTOFF   LPDDR MSD_D3R_PDIFF cell ODT off Receiver
MSD_D3RF2_18_OPEN   DDR2 MSD_D3R_PDIFF_PDQSR Z0=18-Ohm
MSD_D3RF2_40_OPEN   DDR2 MSD_D3R_PDIFF_PDQSR Z0=40-Ohm
MSD_D3RF2_48_OPEN   DDR2 MSD_D3R_PDIFF_PDQSR Z0=48-Ohm
MSD_D3RF2_18_PD344   DDR2 MSD_D3R_PDIFF_PDQSR Z0=18-Ohm
MSD_D3RF2_40_PD344   DDR2 MSD_D3R_PDIFF_PDQSR Z0=40-Ohm
MSD_D3RF2_48_PD344   DDR2 MSD_D3R_PDIFF_PDQSR Z0=48-Ohm
MSD_D3RF2_18_PD393   DDR2 MSD_D3R_PDIFF_PDQSR Z0=18-Ohm
MSD_D3RF2_40_PD393   DDR2 MSD_D3R_PDIFF_PDQSR Z0=40-Ohm
MSD_D3RF2_48_PD393   DDR2 MSD_D3R_PDIFF_PDQSR Z0=48-Ohm
MSD_D3RF2_18_PD458   DDR2 MSD_D3R_PDIFF_PDQSR Z0=18-Ohm
MSD_D3RF2_40_PD458   DDR2 MSD_D3R_PDIFF_PDQSR Z0=40-Ohm
MSD_D3RF2_48_PD458   DDR2 MSD_D3R_PDIFF_PDQSR Z0=48-Ohm
MSD_D3RF2_18_PD500   DDR2 MSD_D3R_PDIFF_PDQSR Z0=18-Ohm
MSD_D3RF2_40_PD500   DDR2 MSD_D3R_PDIFF_PDQSR Z0=40-Ohm
MSD_D3RF2_48_PD500   DDR2 MSD_D3R_PDIFF_PDQSR Z0=48-Ohm
MSD_D3RF2_18_PD550   DDR2 MSD_D3R_PDIFF_PDQSR Z0=18-Ohm
MSD_D3RF2_40_PD550   DDR2 MSD_D3R_PDIFF_PDQSR Z0=40-Ohm
MSD_D3RF2_48_PD550   DDR2 MSD_D3R_PDIFF_PDQSR Z0=48-Ohm
MSD_D3RF2_18_PD611   DDR2 MSD_D3R_PDIFF_PDQSR Z0=18-Ohm
MSD_D3RF2_40_PD611   DDR2 MSD_D3R_PDIFF_PDQSR Z0=40-Ohm
MSD_D3RF2_48_PD611   DDR2 MSD_D3R_PDIFF_PDQSR Z0=48-Ohm
MSD_D3RF2_18_PD688   DDR2 MSD_D3R_PDIFF_PDQSR Z0=18-Ohm
MSD_D3RF2_40_PD688   DDR2 MSD_D3R_PDIFF_PDQSR Z0=40-Ohm
MSD_D3RF2_48_PD688   DDR2 MSD_D3R_PDIFF_PDQSR Z0=48-Ohm
MSD_D3RF2_18_PU344   DDR2 MSD_D3R_PDIFF_PDQSR Z0=18-Ohm
MSD_D3RF2_40_PU344   DDR2 MSD_D3R_PDIFF_PDQSR Z0=40-Ohm
MSD_D3RF2_48_PU344   DDR2 MSD_D3R_PDIFF_PDQSR Z0=48-Ohm
MSD_D3RF2_18_PU393   DDR2 MSD_D3R_PDIFF_PDQSR Z0=18-Ohm
MSD_D3RF2_40_PU393   DDR2 MSD_D3R_PDIFF_PDQSR Z0=40-Ohm
MSD_D3RF2_48_PU393   DDR2 MSD_D3R_PDIFF_PDQSR Z0=48-Ohm
MSD_D3RF2_18_PU458   DDR2 MSD_D3R_PDIFF_PDQSR Z0=18-Ohm
MSD_D3RF2_40_PU458   DDR2 MSD_D3R_PDIFF_PDQSR Z0=40-Ohm
MSD_D3RF2_48_PU458   DDR2 MSD_D3R_PDIFF_PDQSR Z0=48-Ohm
MSD_D3RF2_18_PU500   DDR2 MSD_D3R_PDIFF_PDQSR Z0=18-Ohm
MSD_D3RF2_40_PU500   DDR2 MSD_D3R_PDIFF_PDQSR Z0=40-Ohm
MSD_D3RF2_48_PU500   DDR2 MSD_D3R_PDIFF_PDQSR Z0=48-Ohm
MSD_D3RF2_18_PU550   DDR2 MSD_D3R_PDIFF_PDQSR Z0=18-Ohm
MSD_D3RF2_40_PU550   DDR2 MSD_D3R_PDIFF_PDQSR Z0=40-Ohm
MSD_D3RF2_48_PU550   DDR2 MSD_D3R_PDIFF_PDQSR Z0=48-Ohm
MSD_D3RF2_18_PU611   DDR2 MSD_D3R_PDIFF_PDQSR Z0=18-Ohm
MSD_D3RF2_40_PU611   DDR2 MSD_D3R_PDIFF_PDQSR Z0=40-Ohm
MSD_D3RF2_48_PU611   DDR2 MSD_D3R_PDIFF_PDQSR Z0=48-Ohm
MSD_D3RF2_18_PU688   DDR2 MSD_D3R_PDIFF_PDQSR Z0=18-Ohm
MSD_D3RF2_40_PU688   DDR2 MSD_D3R_PDIFF_PDQSR Z0=40-Ohm
MSD_D3RF2_48_PU688   DDR2 MSD_D3R_PDIFF_PDQSR Z0=48-Ohm
MSD_D3RF2_18_PWRDWN   DDR2 MSD_D3R_PDIFF_PDQSR Z0=18-Ohm
MSD_D3RF2_40_PWRDWN   DDR2 MSD_D3R_PDIFF_PDQSR Z0=40-Ohm
MSD_D3RF2_48_PWRDWN   DDR2 MSD_D3R_PDIFF_PDQSR Z0=48-Ohm
MSD_D3RF3_34_OPEN   DDR3 MSD_D3R_PDIFF_PDQSR cell  Z0=34-Ohm
MSD_D3RF3_40_OPEN   DDR3 MSD_D3R_PDIFF_PDQSR cell  Z0=40-Ohm
MSD_D3RF3_48_OPEN   DDR3 MSD_D3R_PDIFF_PDQSR cell  Z0=48-Ohm
MSD_D3RF3_34_PD344   DDR3 MSD_D3R_PDIFF_PDQSR cell  Z0=34-Ohm
MSD_D3RF3_40_PD344   DDR3 MSD_D3R_PDIFF_PDQSR cell  Z0=40-Ohm
MSD_D3RF3_48_PD344   DDR3 MSD_D3R_PDIFF_PDQSR cell  Z0=48-Ohm
MSD_D3RF3_34_PD393   DDR3 MSD_D3R_PDIFF_PDQSR cell  Z0=34-Ohm
MSD_D3RF3_40_PD393   DDR3 MSD_D3R_PDIFF_PDQSR cell  Z0=40-Ohm
MSD_D3RF3_48_PD393   DDR3 MSD_D3R_PDIFF_PDQSR cell  Z0=48-Ohm
MSD_D3RF3_34_PD458   DDR3 MSD_D3R_PDIFF_PDQSR cell  Z0=34-Ohm
MSD_D3RF3_40_PD458   DDR3 MSD_D3R_PDIFF_PDQSR cell  Z0=40-Ohm
MSD_D3RF3_48_PD458   DDR3 MSD_D3R_PDIFF_PDQSR cell  Z0=48-Ohm
MSD_D3RF3_34_PD500   DDR3 MSD_D3R_PDIFF_PDQSR cell  Z0=34-Ohm
MSD_D3RF3_40_PD500   DDR3 MSD_D3R_PDIFF_PDQSR cell  Z0=40-Ohm
MSD_D3RF3_48_PD500   DDR3 MSD_D3R_PDIFF_PDQSR cell  Z0=48-Ohm
MSD_D3RF3_34_PD550   DDR3 MSD_D3R_PDIFF_PDQSR cell  Z0=34-Ohm
MSD_D3RF3_40_PD550   DDR3 MSD_D3R_PDIFF_PDQSR cell  Z0=40-Ohm
MSD_D3RF3_48_PD550   DDR3 MSD_D3R_PDIFF_PDQSR cell  Z0=48-Ohm
MSD_D3RF3_34_PD611   DDR3 MSD_D3R_PDIFF_PDQSR cell  Z0=34-Ohm
MSD_D3RF3_40_PD611   DDR3 MSD_D3R_PDIFF_PDQSR cell  Z0=40-Ohm
MSD_D3RF3_48_PD611   DDR3 MSD_D3R_PDIFF_PDQSR cell  Z0=48-Ohm
MSD_D3RF3_34_PD688   DDR3 MSD_D3R_PDIFF_PDQSR cell  Z0=34-Ohm
MSD_D3RF3_40_PD688   DDR3 MSD_D3R_PDIFF_PDQSR cell  Z0=40-Ohm
MSD_D3RF3_48_PD688   DDR3 MSD_D3R_PDIFF_PDQSR cell  Z0=48-Ohm
MSD_D3RF3_34_PU344   DDR3 MSD_D3R_PDIFF_PDQSR cell  Z0=34-Ohm
MSD_D3RF3_40_PU344   DDR3 MSD_D3R_PDIFF_PDQSR cell  Z0=40-Ohm
MSD_D3RF3_48_PU344   DDR3 MSD_D3R_PDIFF_PDQSR cell  Z0=48-Ohm
MSD_D3RF3_34_PU393   DDR3 MSD_D3R_PDIFF_PDQSR cell  Z0=34-Ohm
MSD_D3RF3_40_PU393   DDR3 MSD_D3R_PDIFF_PDQSR cell  Z0=40-Ohm
MSD_D3RF3_48_PU393   DDR3 MSD_D3R_PDIFF_PDQSR cell  Z0=48-Ohm
MSD_D3RF3_34_PU458   DDR3 MSD_D3R_PDIFF_PDQSR cell  Z0=34-Ohm
MSD_D3RF3_40_PU458   DDR3 MSD_D3R_PDIFF_PDQSR cell  Z0=40-Ohm
MSD_D3RF3_48_PU458   DDR3 MSD_D3R_PDIFF_PDQSR cell  Z0=48-Ohm
MSD_D3RF3_34_PU500   DDR3 MSD_D3R_PDIFF_PDQSR cell  Z0=34-Ohm
MSD_D3RF3_40_PU500   DDR3 MSD_D3R_PDIFF_PDQSR cell  Z0=40-Ohm
MSD_D3RF3_48_PU500   DDR3 MSD_D3R_PDIFF_PDQSR cell  Z0=48-Ohm
MSD_D3RF3_34_PU550   DDR3 MSD_D3R_PDIFF_PDQSR cell  Z0=34-Ohm
MSD_D3RF3_40_PU550   DDR3 MSD_D3R_PDIFF_PDQSR cell  Z0=40-Ohm
MSD_D3RF3_48_PU550   DDR3 MSD_D3R_PDIFF_PDQSR cell  Z0=48-Ohm
MSD_D3RF3_34_PU611   DDR3 MSD_D3R_PDIFF_PDQSR cell  Z0=34-Ohm
MSD_D3RF3_40_PU611   DDR3 MSD_D3R_PDIFF_PDQSR cell  Z0=40-Ohm
MSD_D3RF3_48_PU611   DDR3 MSD_D3R_PDIFF_PDQSR cell  Z0=48-Ohm
MSD_D3RF3_34_PU688   DDR3 MSD_D3R_PDIFF_PDQSR cell  Z0=34-Ohm
MSD_D3RF3_40_PU688   DDR3 MSD_D3R_PDIFF_PDQSR cell  Z0=40-Ohm
MSD_D3RF3_48_PU688   DDR3 MSD_D3R_PDIFF_PDQSR cell  Z0=48-Ohm
MSD_D3RF3_34_PWRDWN   DDR3 MSD_D3R_PDIFF_PDQSR cell  Z0=34-Ohm
MSD_D3RF3_40_PWRDWN   DDR3 MSD_D3R_PDIFF_PDQSR cell  Z0=40-Ohm
MSD_D3RF3_48_PWRDWN   DDR3 MSD_D3R_PDIFF_PDQSR cell  Z0=48-Ohm
MSD_D3RF3L_34_OPEN   DDR3L MSD_D3R_PDIFF_PDQSR cell  Z0=34-Ohm
MSD_D3RF3L_40_OPEN   DDR3L MSD_D3R_PDIFF_PDQSR cell  Z0=40-Ohm
MSD_D3RF3L_48_OPEN   DDR3L MSD_D3R_PDIFF_PDQSR cell  Z0=48-Ohm
MSD_D3RF3L_34_PD344   DDR3L MSD_D3R_PDIFF_PDQSR cell  Z0=34-Ohm
MSD_D3RF3L_40_PD344   DDR3L MSD_D3R_PDIFF_PDQSR cell  Z0=40-Ohm
MSD_D3RF3L_48_PD344   DDR3L MSD_D3R_PDIFF_PDQSR cell  Z0=48-Ohm
MSD_D3RF3L_34_PD393   DDR3L MSD_D3R_PDIFF_PDQSR cell  Z0=34-Ohm
MSD_D3RF3L_40_PD393   DDR3L MSD_D3R_PDIFF_PDQSR cell  Z0=40-Ohm
MSD_D3RF3L_48_PD393   DDR3L MSD_D3R_PDIFF_PDQSR cell  Z0=48-Ohm
MSD_D3RF3L_34_PD458   DDR3L MSD_D3R_PDIFF_PDQSR cell  Z0=34-Ohm
MSD_D3RF3L_40_PD458   DDR3L MSD_D3R_PDIFF_PDQSR cell  Z0=40-Ohm
MSD_D3RF3L_48_PD458   DDR3L MSD_D3R_PDIFF_PDQSR cell  Z0=48-Ohm
MSD_D3RF3L_34_PD500   DDR3L MSD_D3R_PDIFF_PDQSR cell  Z0=34-Ohm
MSD_D3RF3L_40_PD500   DDR3L MSD_D3R_PDIFF_PDQSR cell  Z0=40-Ohm
MSD_D3RF3L_48_PD500   DDR3L MSD_D3R_PDIFF_PDQSR cell  Z0=48-Ohm
MSD_D3RF3L_34_PD550   DDR3L MSD_D3R_PDIFF_PDQSR cell  Z0=34-Ohm
MSD_D3RF3L_40_PD550   DDR3L MSD_D3R_PDIFF_PDQSR cell  Z0=40-Ohm
MSD_D3RF3L_48_PD550   DDR3L MSD_D3R_PDIFF_PDQSR cell  Z0=48-Ohm
MSD_D3RF3L_34_PD611   DDR3L MSD_D3R_PDIFF_PDQSR cell  Z0=34-Ohm
MSD_D3RF3L_40_PD611   DDR3L MSD_D3R_PDIFF_PDQSR cell  Z0=40-Ohm
MSD_D3RF3L_48_PD611   DDR3L MSD_D3R_PDIFF_PDQSR cell  Z0=48-Ohm
MSD_D3RF3L_34_PD688   DDR3L MSD_D3R_PDIFF_PDQSR cell  Z0=34-Ohm
MSD_D3RF3L_40_PD688   DDR3L MSD_D3R_PDIFF_PDQSR cell  Z0=40-Ohm
MSD_D3RF3L_48_PD688   DDR3L MSD_D3R_PDIFF_PDQSR cell  Z0=48-Ohm
MSD_D3RF3L_34_PU344   DDR3L MSD_D3R_PDIFF_PDQSR cell  Z0=34-Ohm
MSD_D3RF3L_40_PU344   DDR3L MSD_D3R_PDIFF_PDQSR cell  Z0=40-Ohm
MSD_D3RF3L_48_PU344   DDR3L MSD_D3R_PDIFF_PDQSR cell  Z0=48-Ohm
MSD_D3RF3L_34_PU393   DDR3L MSD_D3R_PDIFF_PDQSR cell  Z0=34-Ohm
MSD_D3RF3L_40_PU393   DDR3L MSD_D3R_PDIFF_PDQSR cell  Z0=40-Ohm
MSD_D3RF3L_48_PU393   DDR3L MSD_D3R_PDIFF_PDQSR cell  Z0=48-Ohm
MSD_D3RF3L_34_PU458   DDR3L MSD_D3R_PDIFF_PDQSR cell  Z0=34-Ohm
MSD_D3RF3L_40_PU458   DDR3L MSD_D3R_PDIFF_PDQSR cell  Z0=40-Ohm
MSD_D3RF3L_48_PU458   DDR3L MSD_D3R_PDIFF_PDQSR cell  Z0=48-Ohm
MSD_D3RF3L_34_PU500   DDR3L MSD_D3R_PDIFF_PDQSR cell  Z0=34-Ohm
MSD_D3RF3L_40_PU500   DDR3L MSD_D3R_PDIFF_PDQSR cell  Z0=40-Ohm
MSD_D3RF3L_48_PU500   DDR3L MSD_D3R_PDIFF_PDQSR cell  Z0=48-Ohm
MSD_D3RF3L_34_PU550   DDR3L MSD_D3R_PDIFF_PDQSR cell  Z0=34-Ohm
MSD_D3RF3L_40_PU550   DDR3L MSD_D3R_PDIFF_PDQSR cell  Z0=40-Ohm
MSD_D3RF3L_48_PU550   DDR3L MSD_D3R_PDIFF_PDQSR cell  Z0=48-Ohm
MSD_D3RF3L_34_PU611   DDR3L MSD_D3R_PDIFF_PDQSR cell  Z0=34-Ohm
MSD_D3RF3L_40_PU611   DDR3L MSD_D3R_PDIFF_PDQSR cell  Z0=40-Ohm
MSD_D3RF3L_48_PU611   DDR3L MSD_D3R_PDIFF_PDQSR cell  Z0=48-Ohm
MSD_D3RF3L_34_PU688   DDR3L MSD_D3R_PDIFF_PDQSR cell  Z0=34-Ohm
MSD_D3RF3L_40_PU688   DDR3L MSD_D3R_PDIFF_PDQSR cell  Z0=40-Ohm
MSD_D3RF3L_48_PU688   DDR3L MSD_D3R_PDIFF_PDQSR cell  Z0=48-Ohm
MSD_D3RF3L_34_PWRDWN   DDR3L MSD_D3R_PDIFF_PDQSR cell  Z0=34-Ohm
MSD_D3RF3L_40_PWRDWN   DDR3L MSD_D3R_PDIFF_PDQSR cell  Z0=40-Ohm
MSD_D3RF3L_48_PWRDWN   DDR3L MSD_D3R_PDIFF_PDQSR cell  Z0=48-Ohm
MSD_D3RFL2_34_OPEN   LPDDR2 MSD_D3R_PDIFF_PDQSR cell  Z0=34-Ohm
MSD_D3RFL2_40_OPEN   LPDDR2 MSD_D3R_PDIFF_PDQSR cell  Z0=40-Ohm
MSD_D3RFL2_48_OPEN   LPDDR2 MSD_D3R_PDIFF_PDQSR cell  Z0=48-Ohm
MSD_D3RFL2_60_OPEN   LPDDR2 MSD_D3R_PDIFF_PDQSR cell  Z0=60-Ohm
MSD_D3RFL2_80_OPEN   LPDDR2 MSD_D3R_PDIFF_PDQSR cell  Z0=80-Ohm
MSD_D3RFL_48_OPEN   LPDDR MSD_D3R_PDIFF_PDQSR cell  Z0=48-Ohm
MSD_D3RFL2_34_PD344   LPDDR2 MSD_D3R_PDIFF_PDQSR cell  Z0=34-Ohm
MSD_D3RFL2_40_PD344   LPDDR2 MSD_D3R_PDIFF_PDQSR cell  Z0=40-Ohm
MSD_D3RFL2_48_PD344   LPDDR2 MSD_D3R_PDIFF_PDQSR cell  Z0=48-Ohm
MSD_D3RFL2_60_PD344   LPDDR2 MSD_D3R_PDIFF_PDQSR cell  Z0=60-Ohm
MSD_D3RFL2_80_PD344   LPDDR2 MSD_D3R_PDIFF_PDQSR cell  Z0=80-Ohm
MSD_D3RFL_48_PD344   LPDDR MSD_D3R_PDIFF_PDQSR cell  Z0=48-Ohm
MSD_D3RFL2_34_PD393   LPDDR2 MSD_D3R_PDIFF_PDQSR cell  Z0=34-Ohm
MSD_D3RFL2_40_PD393   LPDDR2 MSD_D3R_PDIFF_PDQSR cell  Z0=40-Ohm
MSD_D3RFL2_48_PD393   LPDDR2 MSD_D3R_PDIFF_PDQSR cell  Z0=48-Ohm
MSD_D3RFL2_60_PD393   LPDDR2 MSD_D3R_PDIFF_PDQSR cell  Z0=60-Ohm
MSD_D3RFL2_80_PD393   LPDDR2 MSD_D3R_PDIFF_PDQSR cell  Z0=80-Ohm
MSD_D3RFL_48_PD393   LPDDR MSD_D3R_PDIFF_PDQSR cell  Z0=48-Ohm
MSD_D3RFL2_34_PD458   LPDDR2 MSD_D3R_PDIFF_PDQSR cell  Z0=34-Ohm
MSD_D3RFL2_40_PD458   LPDDR2 MSD_D3R_PDIFF_PDQSR cell  Z0=40-Ohm
MSD_D3RFL2_48_PD458   LPDDR2 MSD_D3R_PDIFF_PDQSR cell  Z0=48-Ohm
MSD_D3RFL2_60_PD458   LPDDR2 MSD_D3R_PDIFF_PDQSR cell  Z0=60-Ohm
MSD_D3RFL2_80_PD458   LPDDR2 MSD_D3R_PDIFF_PDQSR cell  Z0=80-Ohm
MSD_D3RFL_48_PD458   LPDDR MSD_D3R_PDIFF_PDQSR cell  Z0=48-Ohm
MSD_D3RFL2_34_PD500   LPDDR2 MSD_D3R_PDIFF_PDQSR cell  Z0=34-Ohm
MSD_D3RFL2_40_PD500   LPDDR2 MSD_D3R_PDIFF_PDQSR cell  Z0=40-Ohm
MSD_D3RFL2_48_PD500   LPDDR2 MSD_D3R_PDIFF_PDQSR cell  Z0=48-Ohm
MSD_D3RFL2_60_PD500   LPDDR2 MSD_D3R_PDIFF_PDQSR cell  Z0=60-Ohm
MSD_D3RFL2_80_PD500   LPDDR2 MSD_D3R_PDIFF_PDQSR cell  Z0=80-Ohm
MSD_D3RFL_48_PD500   LPDDR MSD_D3R_PDIFF_PDQSR cell  Z0=48-Ohm
MSD_D3RFL2_34_PD550   LPDDR2 MSD_D3R_PDIFF_PDQSR cell  Z0=34-Ohm
MSD_D3RFL2_40_PD550   LPDDR2 MSD_D3R_PDIFF_PDQSR cell  Z0=40-Ohm
MSD_D3RFL2_48_PD550   LPDDR2 MSD_D3R_PDIFF_PDQSR cell  Z0=48-Ohm
MSD_D3RFL2_60_PD550   LPDDR2 MSD_D3R_PDIFF_PDQSR cell  Z0=60-Ohm
MSD_D3RFL2_80_PD550   LPDDR2 MSD_D3R_PDIFF_PDQSR cell  Z0=80-Ohm
MSD_D3RFL_48_PD550   LPDDR MSD_D3R_PDIFF_PDQSR cell  Z0=48-Ohm
MSD_D3RFL2_34_PD611   LPDDR2 MSD_D3R_PDIFF_PDQSR cell  Z0=34-Ohm
MSD_D3RFL2_40_PD611   LPDDR2 MSD_D3R_PDIFF_PDQSR cell  Z0=40-Ohm
MSD_D3RFL2_48_PD611   LPDDR2 MSD_D3R_PDIFF_PDQSR cell  Z0=48-Ohm
MSD_D3RFL2_60_PD611   LPDDR2 MSD_D3R_PDIFF_PDQSR cell  Z0=60-Ohm
MSD_D3RFL2_80_PD611   LPDDR2 MSD_D3R_PDIFF_PDQSR cell  Z0=80-Ohm
MSD_D3RFL_48_PD611   LPDDR MSD_D3R_PDIFF_PDQSR cell  Z0=48-Ohm
MSD_D3RFL2_34_PD688   LPDDR2 MSD_D3R_PDIFF_PDQSR cell  Z0=34-Ohm
MSD_D3RFL2_40_PD688   LPDDR2 MSD_D3R_PDIFF_PDQSR cell  Z0=40-Ohm
MSD_D3RFL2_48_PD688   LPDDR2 MSD_D3R_PDIFF_PDQSR cell  Z0=48-Ohm
MSD_D3RFL2_60_PD688   LPDDR2 MSD_D3R_PDIFF_PDQSR cell  Z0=60-Ohm
MSD_D3RFL2_80_PD688   LPDDR2 MSD_D3R_PDIFF_PDQSR cell  Z0=80-Ohm
MSD_D3RFL_48_PD688   LPDDR MSD_D3R_PDIFF_PDQSR cell  Z0=48-Ohm
MSD_D3RFL2_34_PU344   LPDDR2 MSD_D3R_PDIFF_PDQSR cell  Z0=34-Ohm
MSD_D3RFL2_40_PU344   LPDDR2 MSD_D3R_PDIFF_PDQSR cell  Z0=40-Ohm
MSD_D3RFL2_48_PU344   LPDDR2 MSD_D3R_PDIFF_PDQSR cell  Z0=48-Ohm
MSD_D3RFL2_60_PU344   LPDDR2 MSD_D3R_PDIFF_PDQSR cell  Z0=60-Ohm
MSD_D3RFL2_80_PU344   LPDDR2 MSD_D3R_PDIFF_PDQSR cell  Z0=80-Ohm
MSD_D3RFL_48_PU344   LPDDR MSD_D3R_PDIFF_PDQSR cell  Z0=48-Ohm
MSD_D3RFL2_34_PU393   LPDDR2 MSD_D3R_PDIFF_PDQSR cell  Z0=34-Ohm
MSD_D3RFL2_40_PU393   LPDDR2 MSD_D3R_PDIFF_PDQSR cell  Z0=40-Ohm
MSD_D3RFL2_48_PU393   LPDDR2 MSD_D3R_PDIFF_PDQSR cell  Z0=48-Ohm
MSD_D3RFL2_60_PU393   LPDDR2 MSD_D3R_PDIFF_PDQSR cell  Z0=60-Ohm
MSD_D3RFL2_80_PU393   LPDDR2 MSD_D3R_PDIFF_PDQSR cell  Z0=80-Ohm
MSD_D3RFL_48_PU393   LPDDR MSD_D3R_PDIFF_PDQSR cell  Z0=48-Ohm
MSD_D3RFL2_34_PU458   LPDDR2 MSD_D3R_PDIFF_PDQSR cell  Z0=34-Ohm
MSD_D3RFL2_40_PU458   LPDDR2 MSD_D3R_PDIFF_PDQSR cell  Z0=40-Ohm
MSD_D3RFL2_48_PU458   LPDDR2 MSD_D3R_PDIFF_PDQSR cell  Z0=48-Ohm
MSD_D3RFL2_60_PU458   LPDDR2 MSD_D3R_PDIFF_PDQSR cell  Z0=60-Ohm
MSD_D3RFL2_80_PU458   LPDDR2 MSD_D3R_PDIFF_PDQSR cell  Z0=80-Ohm
MSD_D3RFL_48_PU458   LPDDR MSD_D3R_PDIFF_PDQSR cell  Z0=48-Ohm
MSD_D3RFL2_34_PU500   LPDDR2 MSD_D3R_PDIFF_PDQSR cell  Z0=34-Ohm
MSD_D3RFL2_40_PU500   LPDDR2 MSD_D3R_PDIFF_PDQSR cell  Z0=40-Ohm
MSD_D3RFL2_48_PU500   LPDDR2 MSD_D3R_PDIFF_PDQSR cell  Z0=48-Ohm
MSD_D3RFL2_60_PU500   LPDDR2 MSD_D3R_PDIFF_PDQSR cell  Z0=60-Ohm
MSD_D3RFL2_80_PU500   LPDDR2 MSD_D3R_PDIFF_PDQSR cell  Z0=80-Ohm
MSD_D3RFL_48_PU500   LPDDR MSD_D3R_PDIFF_PDQSR cell  Z0=48-Ohm
MSD_D3RFL2_34_PU550   LPDDR2 MSD_D3R_PDIFF_PDQSR cell  Z0=34-Ohm
MSD_D3RFL2_40_PU550   LPDDR2 MSD_D3R_PDIFF_PDQSR cell  Z0=40-Ohm
MSD_D3RFL2_48_PU550   LPDDR2 MSD_D3R_PDIFF_PDQSR cell  Z0=48-Ohm
MSD_D3RFL2_60_PU550   LPDDR2 MSD_D3R_PDIFF_PDQSR cell  Z0=60-Ohm
MSD_D3RFL2_80_PU550   LPDDR2 MSD_D3R_PDIFF_PDQSR cell  Z0=80-Ohm
MSD_D3RFL_48_PU550   LPDDR MSD_D3R_PDIFF_PDQSR cell  Z0=48-Ohm
MSD_D3RFL2_34_PU611   LPDDR2 MSD_D3R_PDIFF_PDQSR cell  Z0=34-Ohm
MSD_D3RFL2_40_PU611   LPDDR2 MSD_D3R_PDIFF_PDQSR cell  Z0=40-Ohm
MSD_D3RFL2_48_PU611   LPDDR2 MSD_D3R_PDIFF_PDQSR cell  Z0=48-Ohm
MSD_D3RFL2_60_PU611   LPDDR2 MSD_D3R_PDIFF_PDQSR cell  Z0=60-Ohm
MSD_D3RFL2_80_PU611   LPDDR2 MSD_D3R_PDIFF_PDQSR cell  Z0=80-Ohm
MSD_D3RFL_48_PU611   LPDDR MSD_D3R_PDIFF_PDQSR cell  Z0=48-Ohm
MSD_D3RFL2_34_PU688   LPDDR2 MSD_D3R_PDIFF_PDQSR cell  Z0=34-Ohm
MSD_D3RFL2_40_PU688   LPDDR2 MSD_D3R_PDIFF_PDQSR cell  Z0=40-Ohm
MSD_D3RFL2_48_PU688   LPDDR2 MSD_D3R_PDIFF_PDQSR cell  Z0=48-Ohm
MSD_D3RFL2_60_PU688   LPDDR2 MSD_D3R_PDIFF_PDQSR cell  Z0=60-Ohm
MSD_D3RFL2_80_PU688   LPDDR2 MSD_D3R_PDIFF_PDQSR cell  Z0=80-Ohm
MSD_D3RFL_48_PU688   LPDDR MSD_D3R_PDIFF_PDQSR cell  Z0=48-Ohm
MSD_D3RFL2_34_PWRDWN   LPDDR2 MSD_D3R_PDIFF_PDQSR cell  Z0=34-Ohm
MSD_D3RFL2_40_PWRDWN   LPDDR2 MSD_D3R_PDIFF_PDQSR cell  Z0=40-Ohm
MSD_D3RFL2_48_PWRDWN   LPDDR2 MSD_D3R_PDIFF_PDQSR cell  Z0=48-Ohm
MSD_D3RFL2_60_PWRDWN   LPDDR2 MSD_D3R_PDIFF_PDQSR cell  Z0=60-Ohm
MSD_D3RFL2_80_PWRDWN   LPDDR2 MSD_D3R_PDIFF_PDQSR cell  Z0=80-Ohm
MSD_D3RFL_48_PWRDWN   LPDDR MSD_D3R_PDIFF_PDQSR cell  Z0=48-Ohm
MSD_D3RF2_ODT150_OPEN   DDR2 MSD_D3R_PDIFF_PDQSR cell 150-Ohm ODT Receiver
MSD_D3RF2_ODT50_OPEN   DDR2 MSD_D3R_PDIFF_PDQSR cell 50-Ohm ODT Receiver
MSD_D3RF2_ODT75_OPEN   DDR2 MSD_D3R_PDIFF_PDQSR cell 75-Ohm ODT Receiver
MSD_D3RF2_ODTOFF_OPEN   DDR2 MSD_D3R_PDIFF_PDQSR cell ODT off Receiver
MSD_D3RF2_ODT150_PD344   DDR2 MSD_D3R_PDIFF_PDQSR cell 150-Ohm ODT Receiver
MSD_D3RF2_ODT50_PD344   DDR2 MSD_D3R_PDIFF_PDQSR cell 50-Ohm ODT Receiver
MSD_D3RF2_ODT75_PD344   DDR2 MSD_D3R_PDIFF_PDQSR cell 75-Ohm ODT Receiver
MSD_D3RF2_ODTOFF_PD344   DDR2 MSD_D3R_PDIFF_PDQSR cell ODT off Receiver
MSD_D3RF2_ODT150_PD393   DDR2 MSD_D3R_PDIFF_PDQSR cell 150-Ohm ODT Receiver
MSD_D3RF2_ODT50_PD393   DDR2 MSD_D3R_PDIFF_PDQSR cell 50-Ohm ODT Receiver
MSD_D3RF2_ODT75_PD393   DDR2 MSD_D3R_PDIFF_PDQSR cell 75-Ohm ODT Receiver
MSD_D3RF2_ODTOFF_PD393   DDR2 MSD_D3R_PDIFF_PDQSR cell ODT off Receiver
MSD_D3RF2_ODT150_PD458   DDR2 MSD_D3R_PDIFF_PDQSR cell 150-Ohm ODT Receiver
MSD_D3RF2_ODT50_PD458   DDR2 MSD_D3R_PDIFF_PDQSR cell 50-Ohm ODT Receiver
MSD_D3RF2_ODT75_PD458   DDR2 MSD_D3R_PDIFF_PDQSR cell 75-Ohm ODT Receiver
MSD_D3RF2_ODTOFF_PD458   DDR2 MSD_D3R_PDIFF_PDQSR cell ODT off Receiver
MSD_D3RF2_ODT150_PD500   DDR2 MSD_D3R_PDIFF_PDQSR cell 150-Ohm ODT Receiver
MSD_D3RF2_ODT50_PD500   DDR2 MSD_D3R_PDIFF_PDQSR cell 50-Ohm ODT Receiver
MSD_D3RF2_ODT75_PD500   DDR2 MSD_D3R_PDIFF_PDQSR cell 75-Ohm ODT Receiver
MSD_D3RF2_ODTOFF_PD500   DDR2 MSD_D3R_PDIFF_PDQSR cell ODT off Receiver
MSD_D3RF2_ODT150_PD550   DDR2 MSD_D3R_PDIFF_PDQSR cell 150-Ohm ODT Receiver
MSD_D3RF2_ODT50_PD550   DDR2 MSD_D3R_PDIFF_PDQSR cell 50-Ohm ODT Receiver
MSD_D3RF2_ODT75_PD550   DDR2 MSD_D3R_PDIFF_PDQSR cell 75-Ohm ODT Receiver
MSD_D3RF2_ODTOFF_PD550   DDR2 MSD_D3R_PDIFF_PDQSR cell ODT off Receiver
MSD_D3RF2_ODT150_PD611   DDR2 MSD_D3R_PDIFF_PDQSR cell 150-Ohm ODT Receiver
MSD_D3RF2_ODT50_PD611   DDR2 MSD_D3R_PDIFF_PDQSR cell 50-Ohm ODT Receiver
MSD_D3RF2_ODT75_PD611   DDR2 MSD_D3R_PDIFF_PDQSR cell 75-Ohm ODT Receiver
MSD_D3RF2_ODTOFF_PD611   DDR2 MSD_D3R_PDIFF_PDQSR cell ODT off Receiver
MSD_D3RF2_ODT150_PD688   DDR2 MSD_D3R_PDIFF_PDQSR cell 150-Ohm ODT Receiver
MSD_D3RF2_ODT50_PD688   DDR2 MSD_D3R_PDIFF_PDQSR cell 50-Ohm ODT Receiver
MSD_D3RF2_ODT75_PD688   DDR2 MSD_D3R_PDIFF_PDQSR cell 75-Ohm ODT Receiver
MSD_D3RF2_ODTOFF_PD688   DDR2 MSD_D3R_PDIFF_PDQSR cell ODT off Receiver
MSD_D3RF2_ODT150_PU344   DDR2 MSD_D3R_PDIFF_PDQSR cell 150-Ohm ODT Receiver
MSD_D3RF2_ODT50_PU344   DDR2 MSD_D3R_PDIFF_PDQSR cell 50-Ohm ODT Receiver
MSD_D3RF2_ODT75_PU344   DDR2 MSD_D3R_PDIFF_PDQSR cell 75-Ohm ODT Receiver
MSD_D3RF2_ODTOFF_PU344   DDR2 MSD_D3R_PDIFF_PDQSR cell ODT off Receiver
MSD_D3RF2_ODT150_PU393   DDR2 MSD_D3R_PDIFF_PDQSR cell 150-Ohm ODT Receiver
MSD_D3RF2_ODT50_PU393   DDR2 MSD_D3R_PDIFF_PDQSR cell 50-Ohm ODT Receiver
MSD_D3RF2_ODT75_PU393   DDR2 MSD_D3R_PDIFF_PDQSR cell 75-Ohm ODT Receiver
MSD_D3RF2_ODTOFF_PU393   DDR2 MSD_D3R_PDIFF_PDQSR cell ODT off Receiver
MSD_D3RF2_ODT150_PU458   DDR2 MSD_D3R_PDIFF_PDQSR cell 150-Ohm ODT Receiver
MSD_D3RF2_ODT50_PU458   DDR2 MSD_D3R_PDIFF_PDQSR cell 50-Ohm ODT Receiver
MSD_D3RF2_ODT75_PU458   DDR2 MSD_D3R_PDIFF_PDQSR cell 75-Ohm ODT Receiver
MSD_D3RF2_ODTOFF_PU458   DDR2 MSD_D3R_PDIFF_PDQSR cell ODT off Receiver
MSD_D3RF2_ODT150_PU500   DDR2 MSD_D3R_PDIFF_PDQSR cell 150-Ohm ODT Receiver
MSD_D3RF2_ODT50_PU500   DDR2 MSD_D3R_PDIFF_PDQSR cell 50-Ohm ODT Receiver
MSD_D3RF2_ODT75_PU500   DDR2 MSD_D3R_PDIFF_PDQSR cell 75-Ohm ODT Receiver
MSD_D3RF2_ODTOFF_PU500   DDR2 MSD_D3R_PDIFF_PDQSR cell ODT off Receiver
MSD_D3RF2_ODT150_PU550   DDR2 MSD_D3R_PDIFF_PDQSR cell 150-Ohm ODT Receiver
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| Models and submodels in the file (581): io8_ft_et_fs_1v2 (I/O), io8_ft_et_hs_1v2 (I/O), io8_ft_et_hslv_fs_1v2 (I/O), io8_ft_et_hslv_hs_1v2 (I/O), io8_ft_et_hslv_ls_1v2 (I/O), io8_ft_et_hslv_ms_1v2 (I/O), io8_ft_et_ls_1v2 (I/O), io8_ft_et_ms_1v2 (I/O), io8_ft_fs_1v2 (I/O), io8_ft_hs_1v2 (I/O), io8_ft_hslv_fs_1v2 (I/O), io8_ft_hslv_hs_1v2 (I/O), io8_ft_hslv_ls_1v2 (I/O), io8_ft_hslv_ms_1v2 (I/O), io8_ft_i2c_1v2 (I/O_open_drain), io8_ft_i2c_hslv_1v2 (I/O_open_drain), io8_ft_ls_1v2 (I/O), io8_ft_ms_1v2 (I/O), isudqf_1v2 (Input), io8_ft_et_fs_1v8 (I/O), io8_ft_et_hs_1v8 (I/O), io8_ft_et_hslv_fs_1v8 (I/O), io8_ft_et_hslv_hs_1v8 (I/O), io8_ft_et_hslv_ls_1v8 (I/O), io8_ft_et_hslv_ms_1v8 (I/O), io8_ft_et_ls_1v8 (I/O), io8_ft_et_ms_1v8 (I/O), io8_ft_fs_1v8 (I/O), io8_ft_hs_1v8 (I/O), io8_ft_hslv_fs_1v8 (I/O), io8_ft_hslv_hs_1v8 (I/O), io8_ft_hslv_ls_1v8 (I/O), io8_ft_hslv_ms_1v8 (I/O), io8_ft_i2c_1v8 (I/O_open_drain), io8_ft_i2c_hslv_1v8 (I/O_open_drain), io8_ft_ls_1v8 (I/O), io8_ft_ms_1v8 (I/O), isudqf_1v8 (Input), io8_ft_et_hslv_fs_2v5 (I/O), io8_ft_et_hslv_hs_2v5 (I/O), io8_ft_et_hslv_ls_2v5 (I/O), io8_ft_et_hslv_ms_2v5 (I/O), io8_ft_hslv_fs_2v5 (I/O), io8_ft_hslv_hs_2v5 (I/O), io8_ft_hslv_ls_2v5 (I/O), io8_ft_hslv_ms_2v5 (I/O), io8_ft_i2c_hslv_2v5 (I/O_open_drain), io8_ft_et_fs_3v3 (I/O), io8_ft_et_hs_3v3 (I/O), io8_ft_et_ls_3v3 (I/O), io8_ft_et_ms_3v3 (I/O), io8_ft_fs_3v3 (I/O), io8_ft_hs_3v3 (I/O), io8_ft_i2c_3v3 (I/O_open_drain), io8_ft_ls_3v3 (I/O), io8_ft_ms_3v3 (I/O), io8usb_ft_hs_3v3 (I/O), io8usb_ft_ls_3v3 (I/O), isudqf_3v3 (Input), MSD_D3RF2_18 (I/O), MSD_D3RF2_40 (I/O), MSD_D3RF2_48 (I/O), MSD_D3RF2_ODT150 (Input), MSD_D3RF2_ODT50 (Input), MSD_D3RF2_ODT75 (Input), MSD_D3RF2_ODTOFF (Input), MSD_D3RF3_34 (I/O), MSD_D3RF3_40 (I/O), MSD_D3RF3_48 (I/O), MSD_D3RF3L_34 (I/O), MSD_D3RF3L_40 (I/O), MSD_D3RF3L_48 (I/O), MSD_D3RF3L_ODT120 (Input), MSD_D3RF3L_ODT40 (Input), MSD_D3RF3L_ODT60 (Input), MSD_D3RF3L_ODTOFF (Input), MSD_D3RF3_ODT120 (Input), MSD_D3RF3_ODT40 (Input), MSD_D3RF3_ODT60 (Input), MSD_D3RF3_ODTOFF (Input)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
